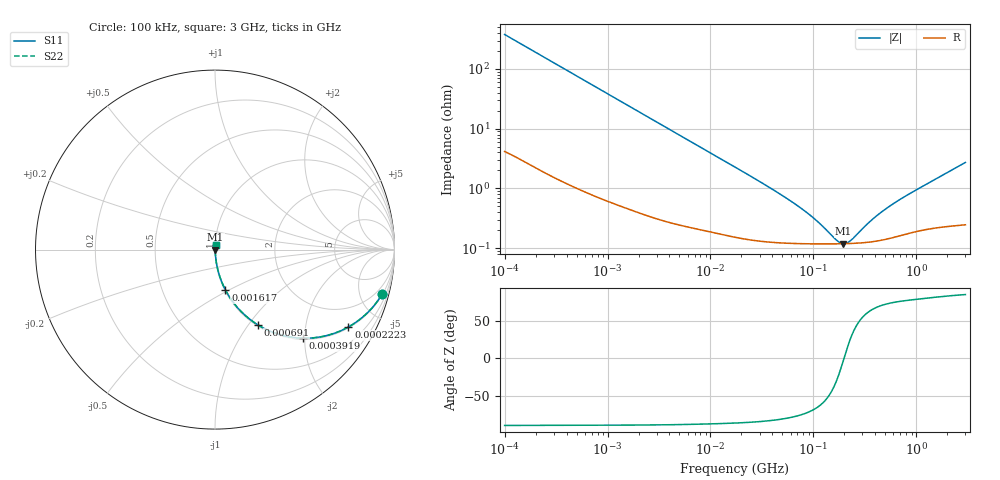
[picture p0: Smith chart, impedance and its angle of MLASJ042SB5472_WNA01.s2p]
! MLASJ042SB5472_WNA01  S-PARAMETER MODEL  ( Standard Model )
! Model Generated by TAIYO YUDEN Corporation (http://www.ty-top.com)
! Version 1.0
! TAIYO YUDEN Control No. 220601
! Copyright(c) 2007 TAIYO YUDEN CO.,LTD. All Rights Reserved.
! Product Description (link to TY-COMPAS)
! https://ds.yuden.co.jp/TYCOMPAS/or/detail?pn=MLASJ042SB5472KWNA01&u=M
! Products Name : Multilayer Ceramic Capacitors
! Characteristics :
!  Capacitance : 4700 [pF] , Rated Voltage : 6.3 [V] , TCC : X5R
!  Case Size : 0.4 x 0.2 / 0.016 x 0.008 [mm/inch] , Thickness : 0.2 / 0.008 [mm/inch]
!  (Conditions: Temperature = 25 [degC] , DC Bias Voltage = 0 [V])
! External Node Assignments :
!  1  o---| |---o  2
! GND o---------o GND
! Frequency Range : 100kHz  -  3GHz  [ 401 STEP ]
# MHZ S RI R 50
! Freq[MHz].  S11 Real  S11 Imag  S21 Real  S21 Imag  S12 Real  S12 Imag  S22 Real  S22 Imag
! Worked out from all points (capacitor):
!   401 points, 100 kHz to 3 GHz, reference 50 ohm
!   read as one part in series: C = 4.19 nF near 105.3 kHz
!   lowest |Z| = 119 mohm at 195.3 MHz (marker M1)
!   series resonance near 198.4 MHz, so ESL is about 150 pH
!   S11 on the Smith chart (normalised r, x): 100 kHz: 1.08, -7.57; 222.3 kHz: 1.04, -3.43; 391.9 kHz: 1.02, -1.95; 691 kHz: 1.02, -1.11; 1.617 MHz: 1.01, -0.48; 3 GHz: 1.00, +0.05
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0.1  0.9324 -0.2456  0.0676 0.2456  0.0676 0.2456  0.9324 -0.2456
0.151038  0.8606 -0.3406  0.1394 0.3406  0.1394 0.3406  0.8606 -0.3406
0.222319  0.7435 -0.4309  0.2565 0.4309  0.2565 0.4309  0.7435 -0.4309
0.302894  0.6123 -0.4812  0.3877 0.4812  0.3877 0.4812  0.6123 -0.4812
0.391939  0.4878 -0.4936  0.5122 0.4936  0.5122 0.4936  0.4878 -0.4936
0.562235  0.3196 -0.4596  0.6804 0.4596  0.6804 0.4596  0.3196 -0.4596
0.690972  0.239 -0.4194  0.761 0.4194  0.761 0.4194  0.239 -0.4194
1.017073  0.1293 -0.3276  0.8707 0.3276  0.8707 0.3276  0.1293 -0.3276
1.61742  0.0578 -0.2241  0.9422 0.2241  0.9422 0.2241  0.0578 -0.2241
3.161081  0.0178 -0.1204  0.9822 0.1204  0.9822 0.1204  0.0178 -0.1204
6.674626  0.00558 -0.0582  0.9944 0.0582  0.9944 0.0582  0.00558 -0.0582
17.7727  0.002 -0.0221  0.998 0.0221  0.998 0.0221  0.002 -0.0221
52.46276  0.00126 -0.00709  0.9987 0.00709  0.9987 0.00709  0.00126 -0.00709
97.38194  0.00119 -0.00312  0.9988 0.00312  0.9988 0.00312  0.00119 -0.00312
167.3121  0.00118 -0.000693  0.9988 0.000693  0.9988 0.000693  0.00118 -0.000693
195.2919  0.00119 -6.43e-05  0.9988 6.43e-05  0.9988 6.43e-05  0.00119 -6.43e-05
210.9903  0.00119 0.000249  0.9988 -0.000249  0.9988 -0.000249  0.00119 0.000249
227.9507  0.0012 0.000564  0.9988 -0.000564  0.9988 -0.000564  0.0012 0.000564
362.5028  0.00128 0.00259  0.9987 -0.00259  0.9987 -0.00259  0.00128 0.00259
547.5153  0.00147 0.00479  0.9985 -0.00479  0.9985 -0.00479  0.00147 0.00479
916.7529  0.0019 0.00847  0.9981 -0.00847  0.9981 -0.00847  0.0019 0.00847
3000  0.00319 0.027  0.9968 -0.027  0.9968 -0.027  0.00319 0.027
